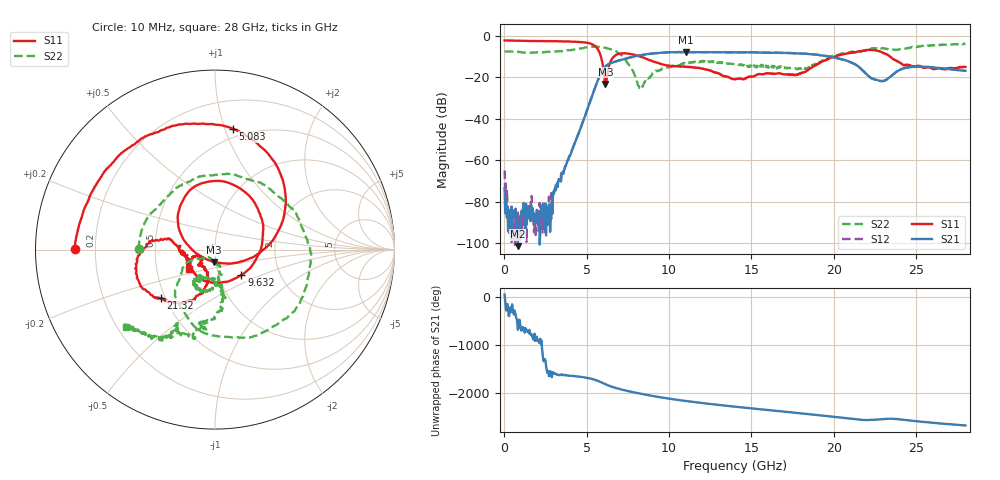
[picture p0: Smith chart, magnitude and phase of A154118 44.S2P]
!  2-Port S-parameters saved by WinCal
! VAR MeasName=S-Parameters (CALIBRATED_DATA) read from VNA (N5230A)
! VAR MeasDate=2015-9-10 14:37:52
! VAR NAME=A154118 44
! VAR FILENAME=A154118 44.S2P
! VAR DATE=2015-9-10 14:37:52
! VAR PHYS_PORTS=1,2
# Hz S DB R 50
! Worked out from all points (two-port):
!   801 points, 10 MHz to 28 GHz, reference 50 ohm
!   highest |S21| = -7.77 dB at 11.03 GHz (marker M1); lowest = -101.5 dB at 814.7 MHz (marker M2)
!   |S21| within 3 dB of the highest: 7.43 GHz to 20.24 GHz (12.81 GHz wide, 92.6 % of centre)
!   lowest |S11| = -23.1 dB at 6.133 GHz (marker M3), VSWR 1.15, Z = 49 - j6.83 ohm
!   |S11| at or under -10 dB: 5.862 GHz to 6.644 GHz (781.6 MHz wide, 12.5 % of centre); 8.257 GHz to 20.06 GHz (11.8 GHz wide, 83.4 % of centre); 23.43 GHz to end of sweep
!   |S22| runs from -25.5 to -3.6 dB; largest |S21 - S12| = 0.0076
!   S11 on the Smith chart (normalised r, x): 10 MHz: 0.12, +0.00; 5.083 GHz: 0.43, +1.07; 9.632 GHz: 1.28, -0.38; 21.32 GHz: 0.48, -0.31; 28 GHz: 0.73, -0.16
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1e7  -2.15 179.6  -73.54 52.9  -64.90 -9.0  -7.50 179.8
2.549125e8  -2.18 176.2  -88.91 -34.5  -91.44 137.2  -7.45 172.1
8.147125e8  -2.30 168.8  -101.54 37.3  -85.30 166.3  -7.62 154.9
2.774012e9  -2.50 142.1  -94.61 -114.0  -86.07 -131.5  -7.66 97.3
4.698325e9  -3.01 98.1  -42.82 125.8  -42.66 125.4  -5.94 12.3
5.083188e9  -3.34 81.5  -34.33 103.4  -34.33 103.2  -5.37 -8.0
5.677975e9  -6.46 33.8  -21.26 43.7  -21.25 43.5  -5.13 -43.6
6.132812e9  -23.14 -94.7  -14.75 -26.1  -14.75 -26.3  -5.71 -70.3
6.797575e9  -8.99 114.3  -12.20 -108.4  -12.21 -108.4  -7.47 -109.2
8.232062e9  -9.90 38.0  -9.34 137.1  -9.31 136.9  -25.29 -129.3
9.351662e9  -13.06 -27.0  -8.21 67.1  -8.17 66.8  -16.91 -78.5
9.631562e9  -13.76 -44.2  -8.03 51.4  -8.01 51.1  -15.62 -83.1
1.103106e10  -14.79 -115.4  -7.77 -18.6  -7.78 -19.3  -13.15 -95.8
1.246555e10  -16.51 -155.4  -7.84 -79.0  -7.83 -79.6  -12.30 -115.1
1.4005e10  -20.94 -153.4  -7.88 -136.8  -7.88 -137.0  -13.72 -124.2
1.592931e10  -18.10 -137.1  -8.05 155.7  -7.98 155.2  -15.16 -114.7
1.869332e10  -15.03 -102.3  -8.82 58.9  -8.83 58.4  -13.96 -84.3
2.131739e10  -7.90 -138.1  -13.72 -40.6  -13.68 -41.3  -7.84 -97.3
2.243699e10  -6.90 -165.9  -20.80 -50.3  -20.93 -51.0  -5.92 -102.5
2.334666e10  -9.53 171.1  -20.27 -29.2  -20.30 -29.9  -6.50 -117.1
2.485112e10  -14.58 -175.6  -14.84 -74.1  -14.91 -74.9  -5.32 -117.0
2.8e10  -14.94 -143.9  -16.84 -170.2  -16.88 -170.9  -3.63 -138.8
